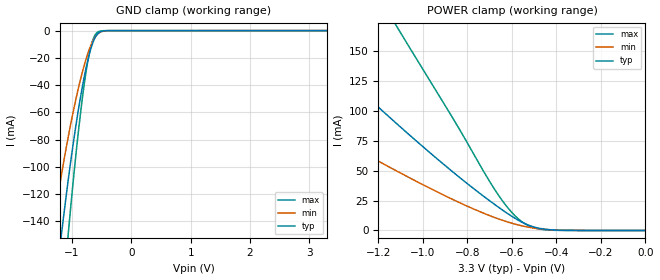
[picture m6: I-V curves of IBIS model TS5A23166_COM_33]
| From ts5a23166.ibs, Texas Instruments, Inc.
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[Model]   TS5A23166_COM_33
Model_type  Terminator
| variable   typ   min   max
C_comp   19.85pF   17.51pF   24.77pF
| C_tri-state   19.85pF   17.51pF   24.77pF
[Temperature Range]   40   100   -40
| Ambient temperature   25   85   -40
[Voltage range]   3.3   3   3.6
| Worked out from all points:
|   GND clamp passes 1 mA (typ) near -0.53 V on its own axis
|   POWER clamp passes 1 mA (typ) near -0.45 V on its own axis
[GND Clamp]
| TS5A23166_COM_33
|   Voltage   I(typ)   I(min)   I(max)
-3.3V     -1.298A    -961.4mA   -1.721A
-1.33V    -208.6mA   -147.2mA   -292.2mA
-1.165V   -144.7mA   -102.5mA   -200.4mA
-1.065V   -109.9mA   -78.27mA   -149.9mA
-1.04V    -101.7mA   -72.58mA   -137.9mA
-895mV    -58.76mA   -42.7mA    -75.15mA
-770mV    -28.86mA   -21.85mA   -32.14mA
-720mV    -19.29mA   -15.13mA   -19.32mA
-665mV    -10.87mA   -9.082mA   -9.046mA
-615mV    -5.489mA   -4.996mA   -3.513mA
-550mV    -1.685mA   -1.792mA   -681.3uA
3.3V      993.7pA    34.74uA    82.97pA
[POWER Clamp]
| TS5A23166_COM_33
|   Voltage   I(typ)   I(min)   I(max)
-3.3V     576.1mA    348.8mA    1.047A
-2.145V   285.6mA    168.5mA    530.7mA
-1.585V   171.2mA    98.86mA    323.8mA
-1.535V   162mA      93.28mA    306.4mA
-1.11V    88.07mA    48.99mA    168.4mA
-880mV    51.2mA     27.2mA     98.38mA
-675mV    21.41mA    10.66mA    33.55mA
-615mV    13.62mA    6.876mA    18.15mA
-565mV    7.919mA    4.324mA    8.735mA
-520mV    4.065mA    2.574mA    3.564mA
-455mV    1.131mA    972.9uA    646.1uA
-48.03fV  993.7pA    7.207nA    109.3pA
